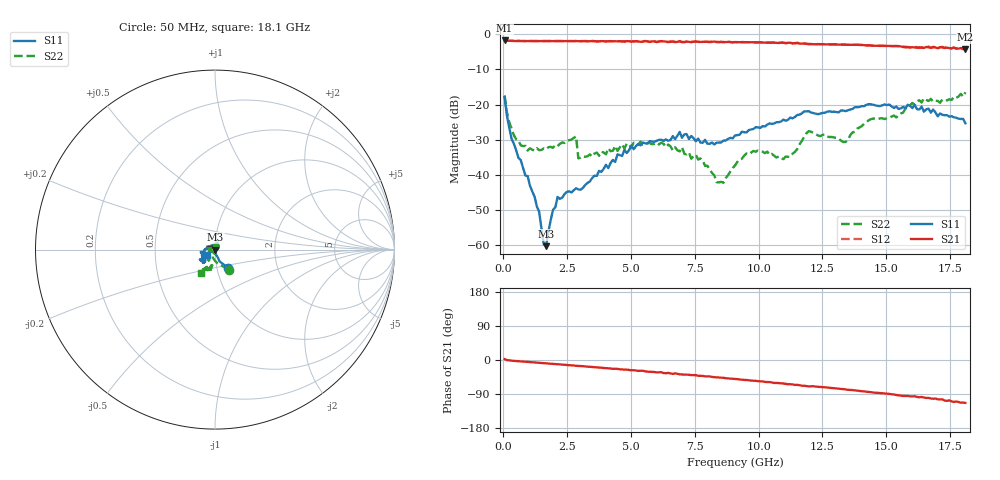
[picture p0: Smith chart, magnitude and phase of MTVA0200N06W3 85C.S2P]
! Network Analyzer HP8720D.06.14 Serial No. US36140669
! 19 Aug 2005  14:33:22
! Frequency  S11  S21  S12  S22
# HZ  S  DB R 50
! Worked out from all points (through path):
!   201 points, 50 MHz to 18.1 GHz, reference 50 ohm
!   highest |S21| = -1.76 dB at 50 MHz (marker M1); lowest = -4.3 dB at 18.1 GHz (marker M2)
!   group delay of S21, straight-line fit = 17.1 ps
!   lowest |S11| = -60.3 dB at 1.675 GHz (marker M3), VSWR 1.00, Z = 50.1 + j0.0297 ohm
!   |S11| at or under -10 dB: start of sweep to end of sweep
!   |S22| runs from -42.3 to -16.5 dB; largest |S21 - S12| = 0.031
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5e7  -17.89 -54.0  -1.76 2.3  -1.78 2.3  -17.41 -55.8
3.2075e8  -29.70 -76.0  -1.88 -1.8  -1.87 -1.7  -26.79 -105.5
6.8175e8  -35.85 -81.6  -1.91 -3.6  -1.92 -3.7  -31.61 -139.7
1.40375e9  -50.57 -58.5  -1.92 -7.4  -1.92 -7.4  -33.01 169.8
1.58425e9  -59.80 -14.7  -1.94 -8.4  -1.93 -8.4  -32.49 158.9
1.6745e9  -60.35 18.0  -1.93 -8.8  -1.93 -8.9  -32.79 152.9
2.12575e9  -46.32 104.3  -1.92 -11.2  -1.93 -11.3  -31.85 126.6
2.84775e9  -43.86 114.8  -1.92 -15.3  -1.93 -15.1  -29.06 100.6
2.938e9  -44.19 -58.2  -1.96 -15.7  -1.93 -15.7  -35.33 108.2
3.1185e9  -43.75 -35.8  -1.94 -16.3  -1.96 -16.5  -34.70 103.3
4.743e9  -32.91 32.3  -2.08 -25.0  -2.04 -25.0  -32.57 71.6
6.09675e9  -30.07 56.4  -2.07 -32.5  -1.99 -32.4  -31.37 46.9
7.54075e9  -30.48 73.6  -2.09 -40.1  -2.02 -41.2  -34.26 39.8
8.353e9  -30.87 118.3  -2.22 -45.8  -2.19 -45.6  -42.10 -12.8
9.075e9  -28.84 153.3  -2.23 -50.0  -2.22 -50.0  -37.37 -89.9
9.797e9  -26.97 169.7  -2.28 -54.6  -2.29 -54.7  -33.24 -98.1
1.1241e10  -23.72 -171.4  -2.42 -63.9  -2.46 -64.2  -34.88 -148.0
1.21435e10  -22.46 -168.4  -2.85 -69.1  -2.82 -69.3  -28.02 154.0
1.3407e10  -21.88 -148.7  -2.98 -77.7  -2.94 -77.4  -30.66 -171.5
1.43095e10  -19.90 -144.2  -3.15 -84.4  -3.12 -84.4  -24.49 -143.3
1.512175e10  -20.02 -143.7  -3.33 -89.7  -3.29 -89.5  -23.79 -128.6
1.81e10  -25.37 -142.8  -4.29 -113.2  -4.22 -114.1  -16.53 -120.6
